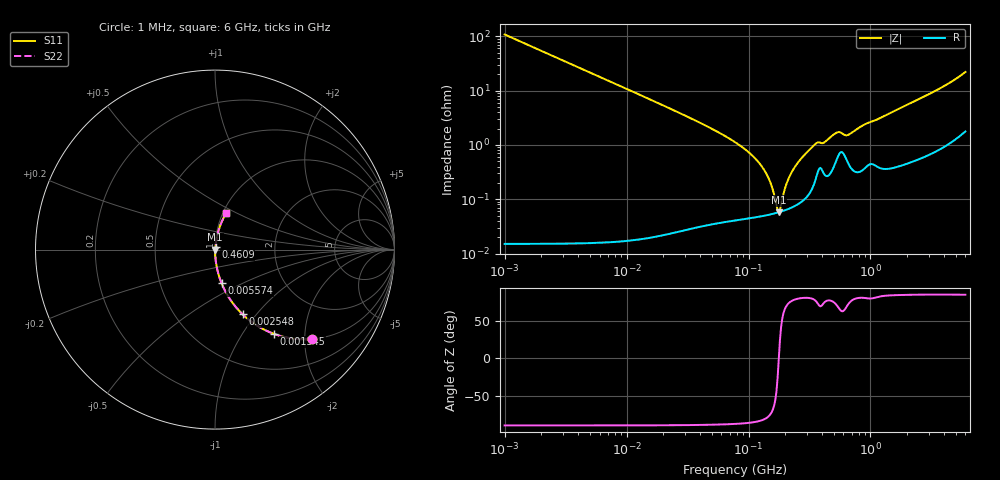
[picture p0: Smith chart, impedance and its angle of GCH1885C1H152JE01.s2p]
!Murata Part Number: GCH1885C1H152JE01
!These Parameters are Measured in Series Mode Connection
!Data Generated on Jun 19, 2026
!  o--ll--o
!Port1  Port2
!  o------o
!Operation Temp=25[degC], DC Bias Voltage=0[V]
!Freq. Start=1000[kHz] Stop=6[GHz] 401[Steps]
# Hz S RI R 50
!Freq.(Hz) S11(Real) S11(Imag) S21(Real) S21(Imag) S12(Real) S12(Imag) S22(Real) S22(Imag)
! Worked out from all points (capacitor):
!   401 points, 1 MHz to 6 GHz, reference 50 ohm
!   read as one part in series: C = 1.47 nF near 1.044 MHz
!   lowest |Z| = 57.5 mohm at 177 MHz (marker M1)
!   series resonance near 177.1 MHz, so ESL is about 550 pH
!   S11 on the Smith chart (normalised r, x): 1 MHz: 1.00, -2.17; 1.545 MHz: 1.00, -1.40; 2.548 MHz: 1.00, -0.85; 5.574 MHz: 1.00, -0.39; 460.9 MHz: 1.01, +0.03; 6 GHz: 1.04, +0.44
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1000000  0.5402 -0.4983  0.4598 0.4983  0.4598 0.4983  0.5402 -0.4983
1544926  0.3299 -0.4701  0.6701 0.4701  0.6701 0.4701  0.3299 -0.4701
2547717  0.1533 -0.3601  0.8467 0.3601  0.8467 0.3601  0.1533 -0.3601
4293785  0.06 -0.2371  0.94 0.2371  0.94 0.2371  0.06 -0.2371
5574230  0.0365 -0.1871  0.9635 0.1871  0.9635 0.1871  0.0365 -0.1871
1.843659e7  0.00357 -0.0578  0.9964 0.0578  0.9964 0.0578  0.00357 -0.0578
7.745967e7  0.000532 -0.0113  0.9995 0.0113  0.9995 0.0113  0.000532 -0.0113
1.050294e8  0.000494 -0.00667  0.9995 0.00667  0.9995 0.00667  0.000494 -0.00667
1.305463e8  0.000504 -0.00379  0.9995 0.00379  0.9995 0.00379  0.000504 -0.00379
1.487431e8  0.000525 -0.00215  0.9995 0.00215  0.9995 0.00215  0.000525 -0.00215
1.694764e8  0.00056 -0.000542  0.9994 0.000542  0.9994 0.000542  0.00056 -0.000542
1.770109e8  0.000575 -6.4e-06  0.9994 6.4e-06  0.9994 6.4e-06  0.000575 -6.4e-06
1.848803e8  0.000592 0.000531  0.9994 -0.000531  0.9994 -0.000531  0.000592 0.000531
2.061188e8  0.000648 0.00189  0.9994 -0.00189  0.9994 -0.00189  0.000648 0.00189
2.248532e8  0.000708 0.00301  0.9993 -0.00301  0.9993 -0.00301  0.000708 0.00301
2.618284e8  0.000869 0.00508  0.9991 -0.00508  0.9991 -0.00508  0.000869 0.00508
3.325952e8  0.00165 0.00899  0.9984 -0.00899  0.9984 -0.00899  0.00165 0.00899
4.608893e8  0.003 0.013  0.997 -0.013  0.997 -0.013  0.003 0.013
5.366786e8  0.00608 0.0159  0.9939 -0.0159  0.9939 -0.0159  0.00608 0.0159
6.527136e8  0.0049 0.0144  0.9951 -0.0144  0.9951 -0.0144  0.0049 0.0144
1.428092e9  0.00506 0.0376  0.9949 -0.0376  0.9949 -0.0376  0.00506 0.0376
6e9  0.0614 0.2033  0.9386 -0.2033  0.9386 -0.2033  0.0614 0.2033
